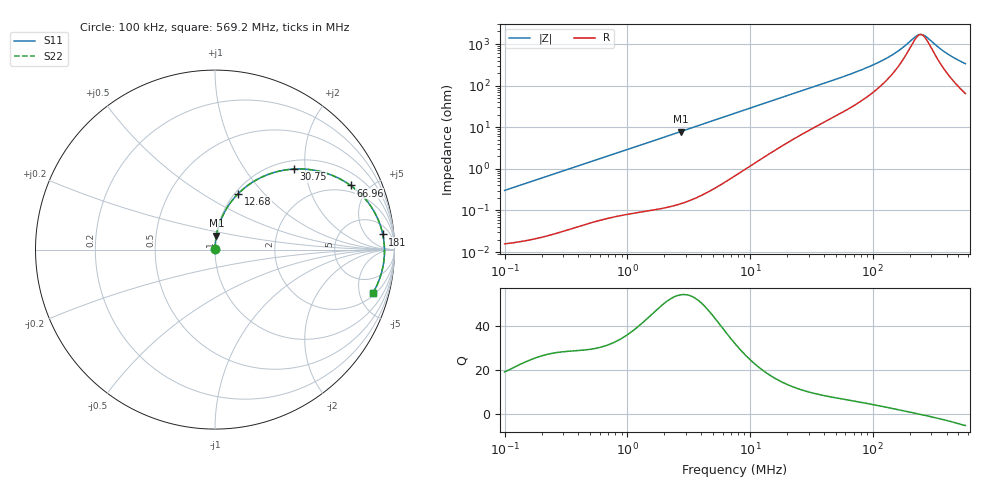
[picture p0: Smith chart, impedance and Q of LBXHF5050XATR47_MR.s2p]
! LBXHF5050XATR47_MR  S-PARAMETER MODEL  ( General Type )
! Model Generated by TAIYO YUDEN Corporation (http://www.ty-top.com)
! Version 1.0
! TAIYO YUDEN Control No. 200511NI43SB-FBB
! Copyright(c) 2020 TAIYO YUDEN CO.,LTD. All Rights Reserved.
! Product Description (link to TY-COMPAS)
! https://ds.yuden.co.jp/TYCOMPAS/or/detail?pn=LBXHF5050XATR47NMR&u=M
! Products Name : Inductors
! Characteristics :
!  Inductance : 0.47 uH , SRF(min) : 180 MHz , DC Resistance(max) : 0.013 Ohm
!  Rated Current : Saturation :11000 mA , Temp Rise : 4100 mA
!  Case Size : 5.0 x 5.0 / 0.197 x 0.197 [mm/inch] , Thickness : 3.1 / 0.122 [mm/inch]
!  (Conditions: Temperature = 25 degC , DC Bias Current/Voltage = 0A / 0V)
! External Node Assignments :
!  1  o---GGG---o  2
! GND o---------o GND
! Frequency Range : 0.1MHz  -  569.217162MHz  [ 402 STEP ]
# MHz S RI R 50
! Freq[MHz].  S11 Real  S11 Imag  S21 Real  S21 Imag  S12 Real  S12 Imag  S22 Real  S22 Imag
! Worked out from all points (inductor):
!   401 points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, 100 kHz to 569.2 MHz, reference 50 ohm
!   read as one part in series: L = 480 nH near 104.4 kHz
!   highest Q = 54.3 at 2.731 MHz (marker M1), where L = 460 nH
!   self-resonance near 245.8 MHz
!   S11 on the Smith chart (normalised r, x): 100 kHz: 1.00, +0.01; 12.68 MHz: 1.04, +0.73; 30.75 MHz: 1.17, +1.73; 66.96 MHz: 1.61, +3.81; 181 MHz: 10, +15; 569.2 MHz: 2.29, -6.61
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0.1  0.000166 0.00303  0.9998 -0.00303  0.9998 -0.00303  0.000166 0.00303
0.425607  0.000593 0.0126  0.9994 -0.0126  0.9994 -0.0126  0.000593 0.0126
1.811416  0.00381 0.0521  0.9962 -0.0521  0.9962 -0.0521  0.00381 0.0521
2.731454  0.00761 0.0782  0.9924 -0.0782  0.9924 -0.0782  0.00761 0.0782
4.689199  0.0208 0.1323  0.9792 -0.1323  0.9792 -0.1323  0.0208 0.1323
7.709517  0.0533 0.2094  0.9467 -0.2094  0.9467 -0.2094  0.0533 0.2094
12.67522  0.1295 0.3118  0.8705 -0.3118  0.8705 -0.3118  0.1295 0.3118
19.11311  0.2455 0.3964  0.7545 -0.3964  0.7545 -0.3964  0.2455 0.3964
30.75188  0.4375 0.4487  0.5625 -0.4487  0.5625 -0.4487  0.4375 0.4487
32.11057  0.4567 0.4495  0.5433 -0.4495  0.5433 -0.4495  0.4567 0.4495
45.37944  0.6084 0.4293  0.3916 -0.4293  0.3916 -0.4293  0.6084 0.4293
66.96482  0.7554 0.3575  0.2446 -0.3575  0.2446 -0.3575  0.7554 0.3575
98.81758  0.8586 0.2553  0.1414 -0.2553  0.1414 -0.2553  0.8586 0.2553
136.6649  0.9105 0.1633  0.0895 -0.1633  0.0895 -0.1633  0.9105 0.1633
181.0105  0.9349 0.0844  0.0651 -0.0844  0.0651 -0.0844  0.9349 0.0844
229.601  0.9436 0.0188  0.0564 -0.0188  0.0564 -0.0188  0.9436 0.0188
244.9844  0.9443 0.000908  0.0557 -0.000908  0.0557 -0.000908  0.9443 0.000908
255.8084  0.9444 -0.011  0.0556 0.011  0.0556 0.011  0.9444 -0.011
278.9122  0.9435 -0.0349  0.0565 0.0349  0.0565 0.0349  0.9435 -0.0349
394.1656  0.9267 -0.1329  0.0733 0.1329  0.0733 0.1329  0.9267 -0.1329
478.8202  0.906 -0.1903  0.094 0.1903  0.094 0.1903  0.906 -0.1903
569.2172  0.8792 -0.2426  0.1208 0.2426  0.1208 0.2426  0.8792 -0.2426
